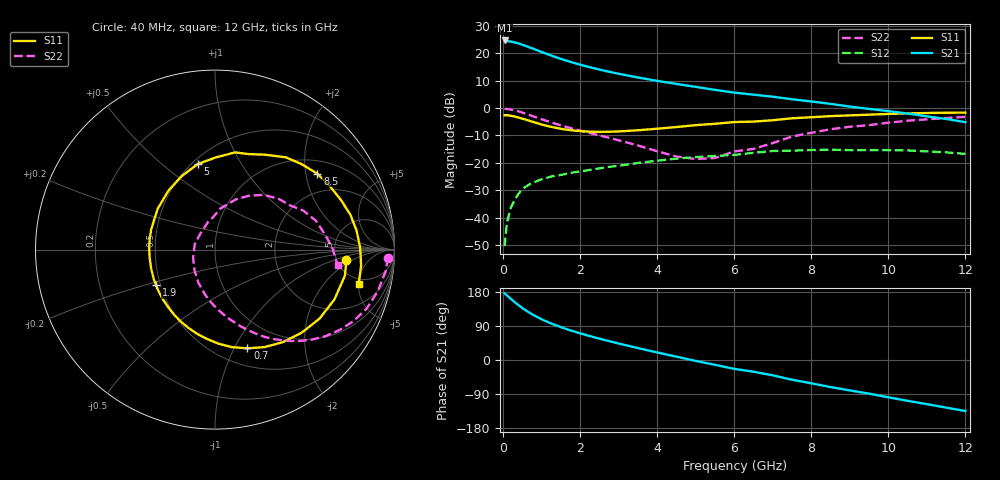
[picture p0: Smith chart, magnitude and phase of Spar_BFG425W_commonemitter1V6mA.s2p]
! Filename: 16bfg425.001
! BFG425W Field C1
! V1=8.393E-001V,V2=1.000E+000V, I1=8.543E-005A, I2=6.000E-003A
# GHz  S  MA  R 50
!  S11  S21  S12  S22
!Freq(GHz)  Mag  Ang  Mag  Ang  Mag  Ang  Mag  Ang
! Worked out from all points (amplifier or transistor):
!   44 points, 40 MHz to 12 GHz, reference 50 ohm
!   highest |S21| = 24.7 dB at 40 MHz (marker M1)
!   |S21| within 3 dB of that: start of sweep to 777.1 MHz
!   unconditionally stable (mu >= 1): 2.233 GHz to end of sweep
!   at 700 MHz: K = 0.39, MSG = 24.9 dB, |S12| = -27.7 dB
!   at 2.4 GHz: K = 1.04, MAG = 17.1 dB, |S12| = -22.3 dB
!   at 12 GHz: K = 1.46, MAG = 1.8 dB, |S12| = -16.8 dB
!   S11 on the Smith chart (normalised r, x): 40 MHz: 6.12, -1.60; 700 MHz: 0.68, -1.13; 1.9 GHz: 0.47, -0.22; 5 GHz: 0.53, +0.67; 8.5 GHz: 1.36, +2.33; 12 GHz: 4.28, -5.02
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0.04  0.735 -4.7  17.09 175.9  0.003 84.3  0.964 -2.7
0.1  0.738 -11.4  16.73 170.5  0.008 84.4  0.959 -7.1
0.2  0.721 -22.6  16.29 161.3  0.015 77.3  0.936 -14.4
0.3  0.698 -33.5  15.76 153.0  0.021 71.4  0.907 -21.2
0.4  0.669 -43.8  15.06 144.8  0.027 65.8  0.868 -27.4
0.5  0.639 -53.9  14.31 137.1  0.033 61.2  0.825 -33.0
0.6  0.609 -63.2  13.48 130.3  0.037 57.1  0.782 -38.1
0.7  0.579 -71.8  12.68 124.0  0.041 53.2  0.738 -42.8
0.9  0.524 -88.0  11.22 112.6  0.047 47.3  0.658 -50.7
1  0.499 -95.4  10.53 107.6  0.05 45.0  0.622 -54.1
1.2  0.46 -109.0  9.33 98.5  0.055 41.0  0.56 -60.3
1.5  0.417 -127.4  7.891 86.8  0.06 36.7  0.481 -68.1
1.9  0.383 -149.0  6.468 73.5  0.068 32.5  0.403 -77.2
2.2  0.371 -163.6  5.669 64.6  0.073 29.7  0.356 -83.8
3  0.373 162.5  4.212 43.5  0.088 22.3  0.257 -102.4
3.5  0.392 144.6  3.604 31.5  0.099 17.0  0.207 -116.5
4.5  0.449 114.6  2.749 8.8  0.119 4.6  0.13 -159.9
5  0.486 101.5  2.428 -2.4  0.127 -3.0  0.117 164.1
6.5  0.564 70.6  1.749 -30.9  0.152 -19.8  0.179 93.9
8.5  0.71 36.6  1.188 -71.4  0.173 -54.6  0.409 48.3
10.5  0.796 7.6  0.791 -107.7  0.168 -87.9  0.585 16.0
12  0.823 -13.3  0.551 -134.7  0.145 -116.5  0.688 -7.2
